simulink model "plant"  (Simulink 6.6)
settings: Solver=FixedStepDiscrete  SolverMode=SingleTasking  StartTime=0.0  StopTime=.999  FixedStep=0.001  RelTol=1e-3
undefined symbols (not defined in the file or in its folder): C, T

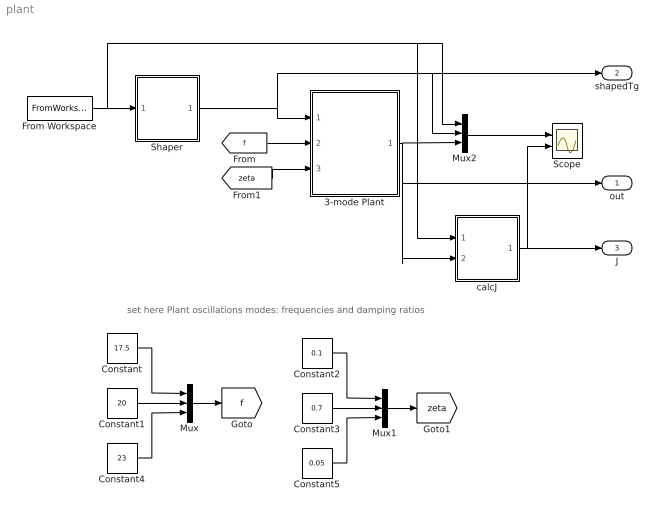
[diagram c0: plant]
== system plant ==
  note: set here Plant oscillations modes: frequencies and damping ratios
  3-mode Plant : Subsystem
  Constant : Constant  Value=17.5
  Constant1 : Constant  Value=20
  Constant2 : Constant  Value=0.1
  Constant3 : Constant  Value=0.7
  Constant4 : Constant  Value=23
  Constant5 : Constant  Value=0.05
  From Workspace : FromWorkspace  VariableName=target  SampleTime=0  Interpolate=off  OutputAfterFinalValue=Holding final value
  Mux : Mux  Inputs=3
  Mux1 : Mux  Inputs=3
  Mux2 : Mux  Inputs=3
  Scope : Scope  NumInputPorts=2
  Shaper : Stateflow chart
  calcJ : Stateflow chart
  out : Outport
  shapedTg : Outport  Port=2
  J : Outport  Port=3
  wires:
  Constant/1 -> Mux/1
  Constant1/1 -> Mux/2
  Constant2/1 -> Mux1/1
  Constant3/1 -> Mux1/2
  Mux/1 -> [f]
  Mux1/1 -> [zeta]
  Constant4/1 -> Mux/3
  Constant5/1 -> Mux1/3
  3-mode Plant/1(out) -> Mux2/3, out/1, calcJ/2(y)
  Mux2/1 -> Scope/1
  [f] -> 3-mode Plant/2(f)
  [zeta] -> 3-mode Plant/3(zeta)
  From Workspace/1 -> Shaper/1(in), Mux2/1, calcJ/1(tg)
  Shaper/1(out) -> 3-mode Plant/1(in), shapedTg/1, Mux2/2
  calcJ/1(J) -> J/1, Scope/2

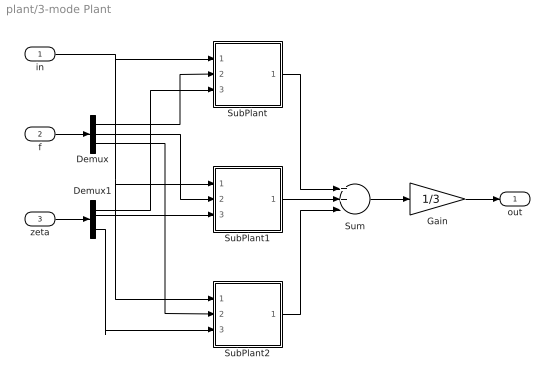
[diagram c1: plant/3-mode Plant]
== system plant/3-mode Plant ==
  in : Inport
  f : Inport  Port=2
  zeta : Inport  Port=3
  Demux : Demux  Outputs=3
  Demux1 : Demux  Outputs=3
  Gain : Gain  Gain=1/3
  SubPlant : Subsystem
  SubPlant1 : Subsystem
  SubPlant2 : Subsystem
  Sum : Sum  Inputs=3
  out : Outport
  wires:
  in/1 -> SubPlant/1(in), SubPlant1/1(in), SubPlant2/1(in)
  f/1 -> Demux/1
  zeta/1 -> Demux1/1
  Demux/1 -> SubPlant/2(f)
  Demux/2 -> SubPlant1/2(f)
  Demux1/1 -> SubPlant/3(zeta)
  SubPlant/1(out) -> Sum/1
  SubPlant1/1(out) -> Sum/2
  Sum/1 -> Gain/1
  Gain/1 -> out/1
  Demux1/2 -> SubPlant1/3(zeta)
  SubPlant2/1(out) -> Sum/3
  Demux/3 -> SubPlant2/2(f)
  Demux1/3 -> SubPlant2/3(zeta)

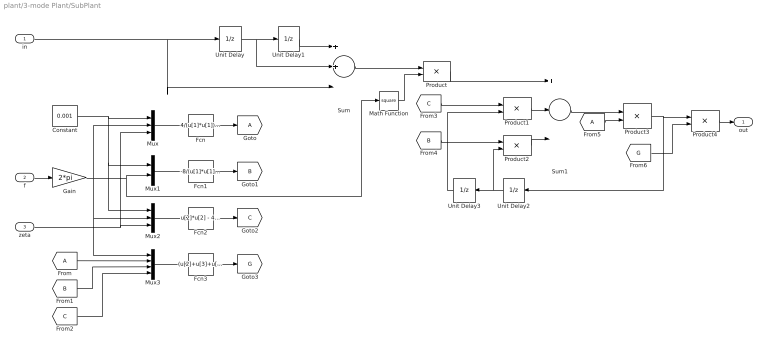
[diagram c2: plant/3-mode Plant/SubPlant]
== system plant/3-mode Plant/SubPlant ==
  in : Inport
  f : Inport  Port=2
  zeta : Inport  Port=3
  Constant : Constant  Value=0.001
  Fcn : Fcn  Expr=4/(u[1]*u[1]) + 4/u[1]*u[2]*u[3] + u[2]*u[2]
  Fcn1 : Fcn  Expr=-8/(u[1]*u[1]) + 2*u[2]*u[2]
  Fcn2 : Fcn  Expr=u[2]*u[2] - 4*u[3]*u[2]/u[1] + 4/(u[1]*u[1])
  Fcn3 : Fcn  Expr=(u[2]+u[3]+u[4]) / (3*u[1]*u[1])
  Gain : Gain  Gain=2*pi
  Math Function : Math  Operator=square
  Mux : Mux  Inputs=3
  Mux1 : Mux  Inputs=2
  Mux2 : Mux  Inputs=3
  Mux3 : Mux
  Product{,1..2,4} (4 alike) : Product
  Product3 : Product  Inputs=*/
  Sum : Sum  Inputs=3
  Sum1 : Sum  Inputs=+--
  Unit Delay : UnitDelay  SampleTime=0.001
  Unit Delay1 : UnitDelay  SampleTime=0.001
  Unit Delay2 : UnitDelay  Orientation=left  SampleTime=0.001
  Unit Delay3 : UnitDelay  Orientation=left  SampleTime=0.001
  out : Outport
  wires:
  Unit Delay1/1 -> Sum/1
  Unit Delay/1 -> Unit Delay1/1, Sum/2
  Sum/1 -> Product/1
  Product/1 -> Sum1/1
  Product1/1 -> Sum1/2
  Product2/1 -> Sum1/3
  Sum1/1 -> Product3/1
  Product3/1 -> Product4/1, Unit Delay2/1
  Unit Delay2/1 -> Unit Delay3/1, Product2/2
  Unit Delay3/1 -> Product1/2
  Mux/1 -> Fcn/1
  Mux1/1 -> Fcn1/1
  Mux2/1 -> Fcn2/1
  Mux3/1 -> Fcn3/1
  in/1 -> Sum/3, Unit Delay/1
  Constant/1 -> Mux/1, Mux1/1, Mux2/1
  f/1 -> Gain/1
  Gain/1 -> Mux1/2, Math Function/1, Mux/2, Mux2/2, Mux3/1
  zeta/1 -> Mux/3, Mux2/3
  Fcn/1 -> [A]
  Fcn1/1 -> [B]
  Fcn2/1 -> [C]
  Fcn3/1 -> [G]
  [A] -> Mux3/2
  [B] -> Mux3/3
  [C] -> Mux3/4
  [C] -> Product1/1
  [B] -> Product2/1
  [A] -> Product3/2
  [G] -> Product4/2
  Math Function/1 -> Product/2
  Product4/1 -> out/1

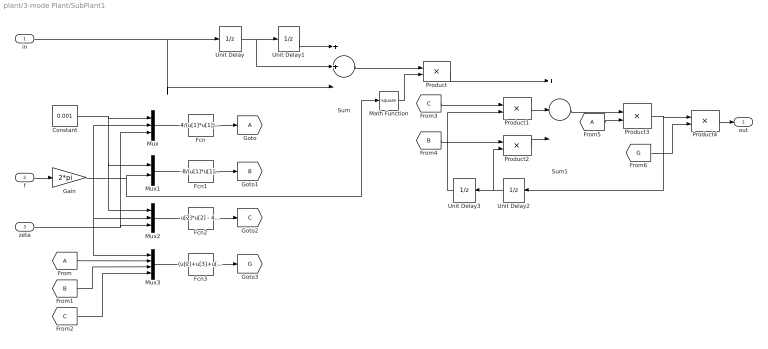
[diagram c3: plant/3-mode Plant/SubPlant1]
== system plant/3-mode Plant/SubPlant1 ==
  in : Inport
  f : Inport  Port=2
  zeta : Inport  Port=3
  Constant : Constant  Value=0.001
  Fcn : Fcn  Expr=4/(u[1]*u[1]) + 4/u[1]*u[2]*u[3] + u[2]*u[2]
  Fcn1 : Fcn  Expr=-8/(u[1]*u[1]) + 2*u[2]*u[2]
  Fcn2 : Fcn  Expr=u[2]*u[2] - 4*u[3]*u[2]/u[1] + 4/(u[1]*u[1])
  Fcn3 : Fcn  Expr=(u[2]+u[3]+u[4]) / (3*u[1]*u[1])
  Gain : Gain  Gain=2*pi
  Math Function : Math  Operator=square
  Mux : Mux  Inputs=3
  Mux1 : Mux  Inputs=2
  Mux2 : Mux  Inputs=3
  Mux3 : Mux
  Product{,1..2,4} (4 alike) : Product
  Product3 : Product  Inputs=*/
  Sum : Sum  Inputs=3
  Sum1 : Sum  Inputs=+--
  Unit Delay : UnitDelay  SampleTime=0.001
  Unit Delay1 : UnitDelay  SampleTime=0.001
  Unit Delay2 : UnitDelay  Orientation=left  SampleTime=0.001
  Unit Delay3 : UnitDelay  Orientation=left  SampleTime=0.001
  out : Outport
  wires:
  Product4/1 -> out/1
  Math Function/1 -> Product/2
  [G] -> Product4/2
  [A] -> Product3/2
  [B] -> Product2/1
  [C] -> Product1/1
  [C] -> Mux3/4
  [B] -> Mux3/3
  [A] -> Mux3/2
  Fcn3/1 -> [G]
  Fcn2/1 -> [C]
  Fcn1/1 -> [B]
  Fcn/1 -> [A]
  zeta/1 -> Mux2/3, Mux/3
  Gain/1 -> Mux3/1, Mux2/2, Mux/2, Math Function/1, Mux1/2
  f/1 -> Gain/1
  Constant/1 -> Mux2/1, Mux1/1, Mux/1
  in/1 -> Unit Delay/1, Sum/3
  Mux3/1 -> Fcn3/1
  Mux2/1 -> Fcn2/1
  Mux1/1 -> Fcn1/1
  Mux/1 -> Fcn/1
  Unit Delay3/1 -> Product1/2
  Unit Delay2/1 -> Product2/2, Unit Delay3/1
  Product3/1 -> Unit Delay2/1, Product4/1
  Sum1/1 -> Product3/1
  Product2/1 -> Sum1/3
  Product1/1 -> Sum1/2
  Product/1 -> Sum1/1
  Sum/1 -> Product/1
  Unit Delay/1 -> Sum/2, Unit Delay1/1
  Unit Delay1/1 -> Sum/1

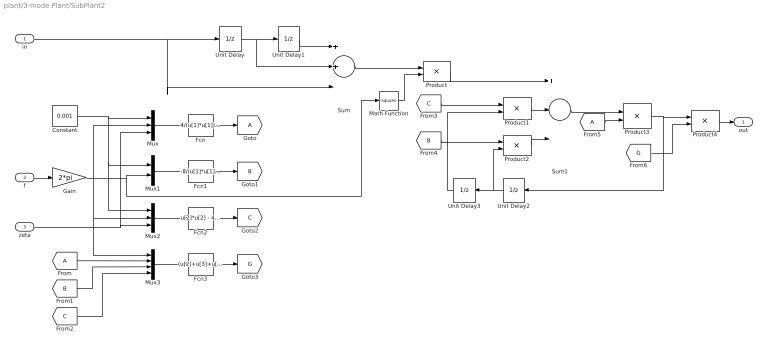
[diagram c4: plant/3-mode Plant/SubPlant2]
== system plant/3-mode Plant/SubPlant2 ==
  in : Inport
  f : Inport  Port=2
  zeta : Inport  Port=3
  Constant : Constant  Value=0.001
  Fcn : Fcn  Expr=4/(u[1]*u[1]) + 4/u[1]*u[2]*u[3] + u[2]*u[2]
  Fcn1 : Fcn  Expr=-8/(u[1]*u[1]) + 2*u[2]*u[2]
  Fcn2 : Fcn  Expr=u[2]*u[2] - 4*u[3]*u[2]/u[1] + 4/(u[1]*u[1])
  Fcn3 : Fcn  Expr=(u[2]+u[3]+u[4]) / (3*u[1]*u[1])
  Gain : Gain  Gain=2*pi
  Math Function : Math  Operator=square
  Mux : Mux  Inputs=3
  Mux1 : Mux  Inputs=2
  Mux2 : Mux  Inputs=3
  Mux3 : Mux
  Product{,1..2,4} (4 alike) : Product
  Product3 : Product  Inputs=*/
  Sum : Sum  Inputs=3
  Sum1 : Sum  Inputs=+--
  Unit Delay : UnitDelay  SampleTime=0.001
  Unit Delay1 : UnitDelay  SampleTime=0.001
  Unit Delay2 : UnitDelay  Orientation=left  SampleTime=0.001
  Unit Delay3 : UnitDelay  Orientation=left  SampleTime=0.001
  out : Outport
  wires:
  Unit Delay1/1 -> Sum/1
  Unit Delay/1 -> Unit Delay1/1, Sum/2
  Sum/1 -> Product/1
  Product/1 -> Sum1/1
  Product1/1 -> Sum1/2
  Product2/1 -> Sum1/3
  Sum1/1 -> Product3/1
  Product3/1 -> Product4/1, Unit Delay2/1
  Unit Delay2/1 -> Unit Delay3/1, Product2/2
  Unit Delay3/1 -> Product1/2
  Mux/1 -> Fcn/1
  Mux1/1 -> Fcn1/1
  Mux2/1 -> Fcn2/1
  Mux3/1 -> Fcn3/1
  in/1 -> Sum/3, Unit Delay/1
  Constant/1 -> Mux/1, Mux1/1, Mux2/1
  f/1 -> Gain/1
  Gain/1 -> Mux1/2, Math Function/1, Mux/2, Mux2/2, Mux3/1
  zeta/1 -> Mux/3, Mux2/3
  Fcn/1 -> [A]
  Fcn1/1 -> [B]
  Fcn2/1 -> [C]
  Fcn3/1 -> [G]
  [A] -> Mux3/2
  [B] -> Mux3/3
  [C] -> Mux3/4
  [C] -> Product1/1
  [B] -> Product2/1
  [A] -> Product3/2
  [G] -> Product4/2
  Math Function/1 -> Product/2
  Product4/1 -> out/1

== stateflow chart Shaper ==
  state DO /
    j = i;
    out = C[0] * in + buf[j];
    buf[j] = 0;
    j = RNG(j+T[0],256);
    buf[j] += C[1] * in;
    j = RNG(j+T[1],256);
    buf[j] += C[2] * in;
    j = RNG(j+T[2],256);
    buf[j] += C[3] * in;
    j = RNG(j+T[3],256);
    buf[j] += C[4] * in;
    j = RNG(j+T[4],256);
    buf[j] += C[5] * in;
    j = RNG(j+T[5],256);
    buf[j] += C[6] * in;
    i = RNG(i+1,256);
  state c = RNG(a,b) [function]
    (default) -> (junction 5)
    (junction 5) -> (junction 6) : {c = a;}
    (junction 5) -> (junction 6) : [a>=b] {c = a-b;}
  (default) -> DO 
  DO  -> DO 

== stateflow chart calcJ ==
  (default) -> (junction 24)
  (junction 24) -> (junction 25) : [(oldy1 < oldy2) && (y > oldy1) || (oldy1 > oldy2) && (y < oldy1)] {err = tg - y; J = J + err * err / 2;}
  (junction 24) -> (junction 25)
  (junction 25) -> (junction 26)
  (junction 25) -> (junction 26) : [y != oldy1] {oldy2 = oldy1; oldy1 = y;}
